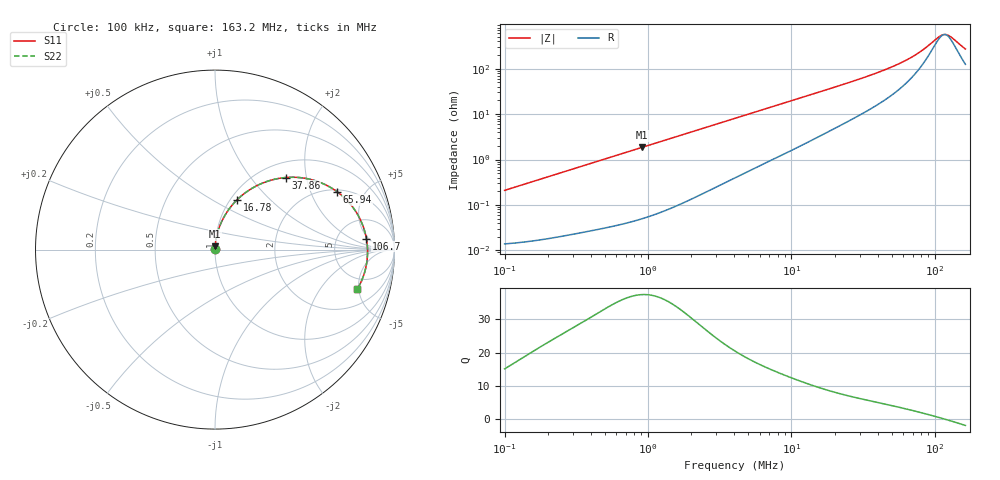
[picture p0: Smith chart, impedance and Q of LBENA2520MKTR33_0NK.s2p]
! LBENA2520MKTR33_0NK  S-PARAMETER MODEL  ( General Type )
! Model Generated by TAIYO YUDEN Corporation (http://www.ty-top.com)
! Version 1.0
! TAIYO YUDEN Control No. 220120
! Copyright(c) 2022 TAIYO YUDEN CO.,LTD. All Rights Reserved.
! Product Description (link to TY-COMPAS)
! https://ds.yuden.co.jp/TYCOMPAS/or/detail?pn=LBENA2520MKTR33M0NK&u=M
! Products Name : Inductors
! Characteristics :
!  Inductance : 0.33 uH , SRF(min) : -Hz , DC Resistance(max) : 0.015 Ohm
!  Rated Current : Saturation :7000 mA , Temp Rise : 5600 mA
!  Case Size : 2.5 x 2.0 / 0.098 x 0.079 [mm/inch] , Thickness : 1.2 / 0.047 [mm/inch]
!  (Conditions: Temperature = 25 degC , DC Bias Current/Voltage = 0A / 0V)
! External Node Assignments :
!  1  o---GGG---o  2
! GND o---------o GND
! Frequency Range : 0.1MHz  -  163.203978MHz  [ 402 STEP ]
# MHz S RI R 50
! Freq[MHz].  S11 Real  S11 Imag  S21 Real  S21 Imag  S12 Real  S12 Imag  S22 Real  S22 Imag
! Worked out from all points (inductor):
!   401 points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, 100 kHz to 163.2 MHz, reference 50 ohm
!   read as one part in series: L = 332 nH near 103.8 kHz
!   highest Q = 37.4 at 903.2 kHz (marker M1), where L = 325 nH
!   self-resonance near 116.7 MHz
!   S11 on the Smith chart (normalised r, x): 100 kHz: 1.00, +0.00; 16.78 MHz: 1.07, +0.65; 37.86 MHz: 1.29, +1.52; 65.94 MHz: 2.10, +3.13; 106.7 MHz: 10, +4; 163.2 MHz: 3.50, -4.81
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0.1  0.000143 0.00209  0.9999 -0.00209  0.9999 -0.00209  0.000143 0.00209
0.345249  0.000297 0.00712  0.9997 -0.00712  0.9997 -0.00712  0.000297 0.00712
0.903207  0.000833 0.0184  0.9992 -0.0184  0.9992 -0.0184  0.000833 0.0184
1.191969  0.00125 0.0243  0.9987 -0.0243  0.9987 -0.0243  0.00125 0.0243
2.319586  0.00386 0.0468  0.9961 -0.0468  0.9961 -0.0468  0.00386 0.0468
4.115259  0.0108 0.0814  0.9892 -0.0814  0.9892 -0.0814  0.0108 0.0814
8.310107  0.0371 0.1561  0.9629 -0.1561  0.9629 -0.1561  0.0371 0.1561
13.94754  0.0902 0.2413  0.9098 -0.2413  0.9098 -0.2413  0.0902 0.2413
16.78093  0.1222 0.2768  0.8778 -0.2768  0.8778 -0.2768  0.1222 0.2768
25.20671  0.2284 0.3538  0.7716 -0.3538  0.7716 -0.3538  0.2284 0.3538
37.86312  0.3929 0.4015  0.6071 -0.4015  0.6071 -0.4015  0.3929 0.4015
48.15376  0.5148 0.3949  0.4852 -0.3949  0.4852 -0.3949  0.5148 0.3949
56.87437  0.6038 0.3667  0.3962 -0.3667  0.3962 -0.3667  0.6038 0.3667
65.94338  0.6804 0.3224  0.3196 -0.3224  0.3196 -0.3224  0.6804 0.3224
73.68213  0.7329 0.277  0.2671 -0.277  0.2671 -0.277  0.7329 0.277
82.32906  0.7783 0.2215  0.2217 -0.2215  0.2217 -0.2215  0.7783 0.2215
106.6593  0.8436 0.0616  0.1564 -0.0616  0.1564 -0.0616  0.8436 0.0616
114.8487  0.8495 0.0111  0.1505 -0.0111  0.1505 -0.0111  0.8495 0.0111
123.6669  0.849 -0.04  0.151 0.04  0.151 0.04  0.849 -0.04
133.1621  0.8423 -0.0908  0.1577 0.0908  0.1577 0.0908  0.8423 -0.0908
157.2777  0.8048 -0.1995  0.1952 0.1995  0.1952 0.1995  0.8048 -0.1995
163.204  0.7925 -0.2218  0.2075 0.2218  0.2075 0.2218  0.7925 -0.2218
